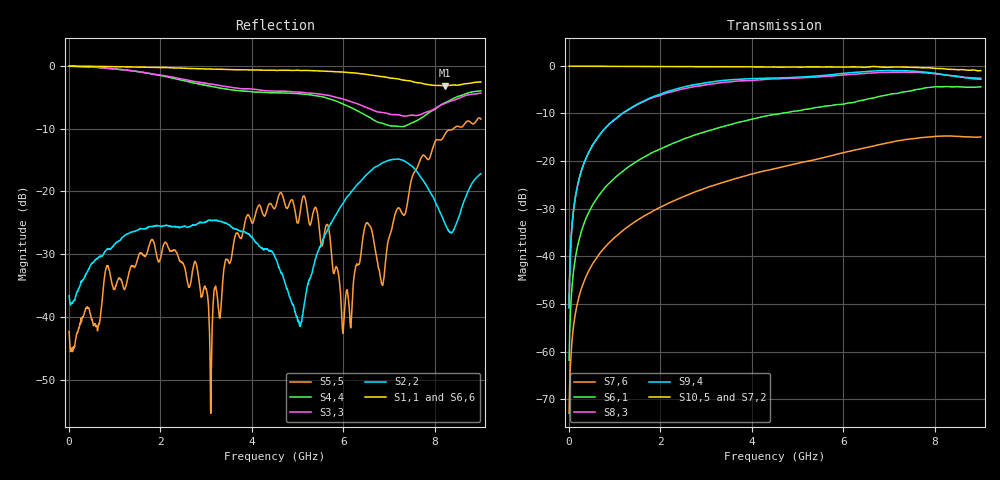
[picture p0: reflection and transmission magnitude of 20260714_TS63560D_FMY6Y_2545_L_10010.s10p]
# GHz S DB R 50
! CMT, SN0916, 25263762, 26.7.0
! Date: 15.07.2026 13:42:28
! Data: Format
! Freq S1.1:dB/Ang S1.2:dB/Ang S1.3:dB/Ang S1.4:dB/Ang S1.5:dB/Ang S1.6:dB/Ang S1.7:dB/Ang S1.8:dB/Ang S1.9:dB/Ang S1.10:dB/Ang
!  S2.1:dB/Ang S2.2:dB/Ang S2.3:dB/Ang S2.4:dB/Ang S2.5:dB/Ang S2.6:dB/Ang S2.7:dB/Ang S2.8:dB/Ang S2.9:dB/Ang S2.10:dB/Ang
!  S3.1:dB/Ang S3.2:dB/Ang S3.3:dB/Ang S3.4:dB/Ang S3.5:dB/Ang S3.6:dB/Ang S3.7:dB/Ang S3.8:dB/Ang S3.9:dB/Ang S3.10:dB/Ang
!  S4.1:dB/Ang S4.2:dB/Ang S4.3:dB/Ang S4.4:dB/Ang S4.5:dB/Ang S4.6:dB/Ang S4.7:dB/Ang S4.8:dB/Ang S4.9:dB/Ang S4.10:dB/Ang
!  S5.1:dB/Ang S5.2:dB/Ang S5.3:dB/Ang S5.4:dB/Ang S5.5:dB/Ang S5.6:dB/Ang S5.7:dB/Ang S5.8:dB/Ang S5.9:dB/Ang S5.10:dB/Ang
!  S6.1:dB/Ang S6.2:dB/Ang S6.3:dB/Ang S6.4:dB/Ang S6.5:dB/Ang S6.6:dB/Ang S6.7:dB/Ang S6.8:dB/Ang S6.9:dB/Ang S6.10:dB/Ang
!  S7.1:dB/Ang S7.2:dB/Ang S7.3:dB/Ang S7.4:dB/Ang S7.5:dB/Ang S7.6:dB/Ang S7.7:dB/Ang S7.8:dB/Ang S7.9:dB/Ang S7.10:dB/Ang
!  S8.1:dB/Ang S8.2:dB/Ang S8.3:dB/Ang S8.4:dB/Ang S8.5:dB/Ang S8.6:dB/Ang S8.7:dB/Ang S8.8:dB/Ang S8.9:dB/Ang S8.10:dB/Ang
!  S9.1:dB/Ang S9.2:dB/Ang S9.3:dB/Ang S9.4:dB/Ang S9.5:dB/Ang S9.6:dB/Ang S9.7:dB/Ang S9.8:dB/Ang S9.9:dB/Ang S9.10:dB/Ang
!  S10.1:dB/Ang S10.2:dB/Ang S10.3:dB/Ang S10.4:dB/Ang S10.5:dB/Ang S10.6:dB/Ang S10.7:dB/Ang S10.8:dB/Ang S10.9:dB/Ang S10.10:dB/Ang
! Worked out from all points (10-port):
!   2001 points, 10 MHz to 9 GHz, reference 50 ohm
!   strongest paths, dB at 10 MHz, 2.257 GHz, 4.505 GHz, 6.753 GHz, 9 GHz:
!     S10,5: -0.1, -0.2, -0.2, -0.2, -1.0
!     S7,2: -0.1, -0.2, -0.3, -0.6, -0.6
!     S9,4: -50.8, -5.1, -2.5, -1.0, -2.8
!     S8,3: -50.7, -5.4, -2.7, -1.4, -2.6
!     S6,1: -61.8, -16.4, -10.2, -6.5, -4.4
!     S7,6: -73.0, -28.5, -21.6, -16.6, -14.9
!   lowest |S11| = -3.1 dB at 8.213 GHz (marker M1), VSWR 5.61, Z = 11 - j23.8 ohm
!   |S11| at or under -10 dB: nowhere
